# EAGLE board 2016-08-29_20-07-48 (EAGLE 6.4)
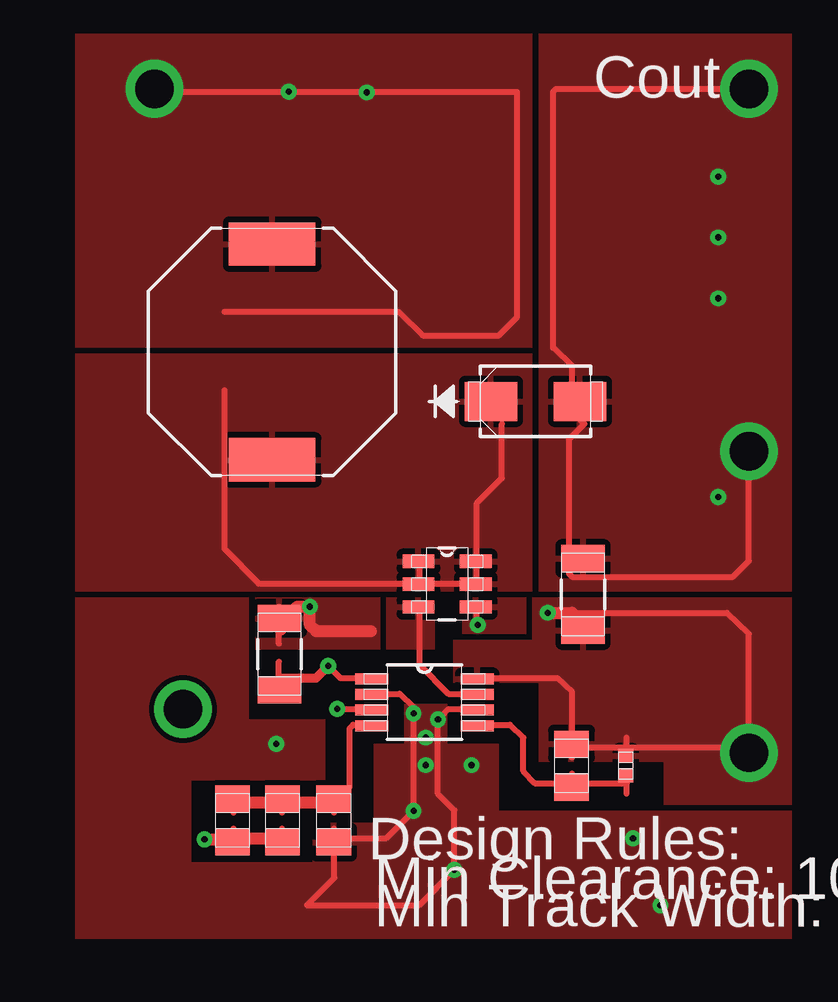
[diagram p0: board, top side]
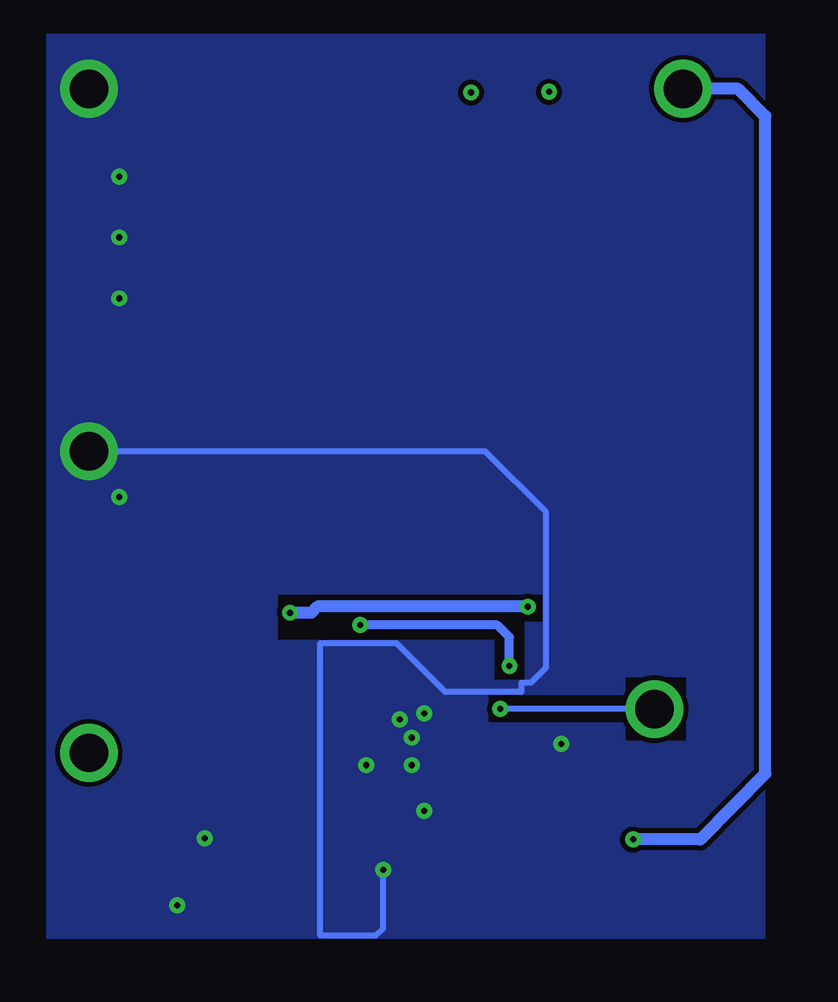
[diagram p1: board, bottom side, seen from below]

No outline drawn. Coordinates in mm, seen from the top.
Copper layers ((1*2)+(15*16)): TOP / INTERNAL1 / layer 15 / BOTTOM

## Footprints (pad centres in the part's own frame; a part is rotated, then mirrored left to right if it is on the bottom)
0805 = smd 1.118 x 1.448: 1 -0.902,0; 2 0.902,0
1206 = smd 1.118 x 1.803: 1 -1.499,0; 2 1.499,0
SMA = smd 2.184 x 1.626: 1 -1.854,0; 2 1.854,0
TP-1502 = drill 0.813 round: 1 0,0
SRU1038 = smd 1.803 x 3.607: 1 -4.496,0; 2 4.496,0
SOT-23-6 = smd 1.321 x 0.559: 1 -1.194,0.95; 2 -1.194,0; 3 -1.194,-0.95; 4 1.194,-0.95; 5 1.194,0; 6 1.194,0.95
0402 = smd 0.559 x 0.61: 1 -0.419,0; 2 0.419,0
MUA08A = smd 1.372 x 0.457: 1 -2.197,0.975; 2 -2.197,0.325; 3 -2.197,-0.325; 4 -2.197,-0.975; 5 2.197,-0.975; 6 2.197,-0.325; 7 2.197,0.325; 8 2.197,0.975

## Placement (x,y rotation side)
Cadj  [0805]  46.96,33.25 270 top
Cff  [0805]  32.84,30.96 90 top
Cin  [1206]  47.45,40.39 90 top
D1  [SMA]  45.47,48.44 0 top
GND  [TP-1502]  54.31,46.33 270 top
GND1  [TP-1502]  54.31,61.42 270 top
L1  [SRU1038]  34.49,50.5 90 top
M1  [SOT-23-6]  41.78,40.82 0 top
NC1  [TP-1502]  30.73,35.56 270 top
Radj  [0402]  49.23,33.25 270 top
Rfbb  [0805]  37.06,30.96 270 top
Rfbt  [0805]  34.92,30.96 90 top
Rsns  [1206]  34.8,37.9 90 top
U1  [MUA08A]  40.84,35.89 0 top
VIN  [TP-1502]  54.31,33.73 270 top
VOUT  [TP-1502]  29.54,61.42 270 top

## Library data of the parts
Cadj = ultra-librarian; RefDes: Cadj; Type: CL21C102JBCNFNC
Cff = ultra-librarian; RefDes: Cff; Type: CL21C331JBANFNC
Cin = ultra-librarian; RefDes: Cin; Type: GRM31CR71H475KA12L
D1 = ultra-librarian; RefDes: D1; Type: B340A-13-F
GND = ultra-librarian; RefDes: GND; Type: TP-1502
GND1 = ultra-librarian; RefDes: GND1; Type: TP-1502
L1 = ultra-librarian; RefDes: L1; Type: SRU1038-100Y
M1 = ultra-librarian; RefDes: M1; Type: FDC5614P
NC1 = ultra-librarian; RefDes: NC1; Type: TP-1502
Radj = ultra-librarian; RefDes: Radj; Type: CRCW040266K5FKED
Rfbb = ultra-librarian; RefDes: Rfbb; Type: ERJ-6ENF4322V
Rfbt = ultra-librarian; RefDes: Rfbt; Type: ERJ-6ENF4322V
Rsns = ultra-librarian; RefDes: Rsns; Type: CSR1206FK20L0
U1 = ultra-librarian; RefDes: U1; Type: LM3485MM/NOPB
VIN = ultra-librarian; RefDes: VIN; Type: TP-1502
VOUT = ultra-librarian; RefDes: VOUT; Type: TP-1502

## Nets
0: Cin.2 D1.2 GND1.1 GND.1 Rfbb.2 U1.2 U1.6
1: Cff.2 Rfbb.1 Rfbt.2 U1.4
2: Cadj.1 Cin.1 Radj.1 Rsns.2 U1.8 VIN.1
3: Cadj.2 Radj.2 U1.5
4: D1.1 L1.1 M1.1 M1.2 M1.5 M1.6
5: M1.4 Rsns.1 U1.1
6: Cff.1 L1.2 Rfbt.1 VOUT.1
7: M1.3 U1.7
8: NC1.1 U1.3

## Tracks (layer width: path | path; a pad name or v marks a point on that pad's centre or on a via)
0  (via drill 0.25 pad 0.56, 1.6 pad 2.21)
  TOP 0.254: v54.36,61.47 46.33,61.47 46.2,61.34 46.2,50.67 46.99,49.91 46.99,48.01 47.5,47.5 46.86,46.86 46.86,41.25 46.99,41.12 53.7,41.12 54.36,41.78 v54.36,46.35 | 38.73,36.25 39.8,36.25 40.39,35.69 v40.39,35.43 v40.39,31.37 39.24,30.23 37.08,30.23 37.08,28.57 35.94,27.43 40.62,27.43 v42.09,28.91 42.09,31.39 41.4,32.08 v41.4,35.18 | 43.03,35.61 41.83,35.61 41.53,35.31 41.53,35.18 | 37.07,29.79 37.07,30.63
  BOTTOM 0.254: v42.09,28.91 42.09,26.47 42.42,26.16 44.7,26.16 44.7,38.35 41.53,38.35 39.5,36.32 36.32,36.32 36.32,36.7 35.94,36.7 35.31,37.34 35.31,43.81 37.85,46.35 v54.36,46.35
  other vias: 53.09,57.81 53.09,55.27 53.09,52.73 53.09,44.45 50.67,27.43 34.67,34.16 40.89,33.27 49.53,30.23 42.8,33.27 40.89,34.42
  pour BOTTOM: 26.16,63.75 56.13,63.75 56.13,26.04 44.7,26.04 44.7,38.48 46.48,38.48 46.48,40.39 35.43,40.39 35.43,39.24 36.2,39.24 36.2,36.2 35.43,36.2 32,36.2 32,36.96 29.46,36.96 29.46,34.29 32,34.29 32,35.05 37.72,35.05 37.72,36.2 36.32,36.2 36.32,36.83 37.47,36.83 37.47,38.48 44.58,38.48 44.58,26.04 26.16,26.04
  pour TOP: 33.53,40.26 26.29,40.26 26.29,26.04 56.13,26.04 56.13,31.37 43.94,31.37 43.94,34.16 41.78,34.16 41.78,35.81 40.01,35.81 40.01,34.16 38.73,34.16 38.73,30.86 36.2,30.86 36.2,29.21 31.11,29.21 31.11,32.64 36.7,32.64 36.7,35.18 33.53,35.18
  pour TOP: 45.59,63.75 45.59,40.51 56.13,40.51 56.13,63.75
1
  TOP 0.254: 38.73,34.95 37.87,34.95 37.72,34.8 37.72,32.36 37.08,31.73 | 32.88,31.29 32.88,32.13 | 34.91,31.29 34.91,32.13 | 37.07,31.29 37.07,32.13
  TOP 0.508: 37.08,31.73 34.92,31.73 32.89,31.73
2  (via drill 0.25 pad 0.56, 1.6 pad 2.21)
  TOP 0.254: 46.99,39.62 53.44,39.62 54.36,38.73 v54.36,33.78 54.1,34.01 49.28,34.01 46.99,34.01 46.99,36.32 46.38,36.91 43.03,36.91 43.05,36.91 | 34.77,38.33 34.77,39.88 | 49.26,33.58 49.26,34.42 | 46.98,33.58 46.98,34.42 | v45.97,39.62
  TOP 0.508: 38.61,38.86 36.32,38.86 36.07,39.12 v36.07,39.88 35.56,39.88 34.85,39.17 34.85,38.91 | v45.97,39.62 46.99,39.62
  BOTTOM 0.508: v36.07,39.88 44.83,39.88 45.09,39.62 v45.97,39.62
  pour TOP (rank 3): 45.59,33.4 45.59,36.7 42.04,36.7 42.04,38.48 45.34,38.48 45.34,40.26 56.13,40.26 56.13,31.62 50.8,31.62 50.8,33.4
  pour TOP (rank 5): 33.78,40.26 38.99,40.26 38.99,38.1 33.78,38.1
3
  TOP 0.254: 49.28,32.51 46.99,32.51 45.44,32.51 44.96,33.02 44.96,34.42 44.4,34.95 43.03,34.95 | 49.26,32.08 49.26,32.92 | 46.98,32.08 46.98,32.92
4
  TOP 0.254: 32.51,48.9 32.51,42.29 33.93,40.84 40.64,40.84 | 40.64,40.84 40.64,41.78 | 40.64,40.84 43.03,40.84 | 44.07,47.5 44.07,45.24 43.03,44.2 43.03,40.89 | 42.65,41.77 43.38,41.77 | 42.65,40.83 43.38,40.83 | 40.26,40.83 41,40.83 | 40.26,41.77 41,41.77
  pour TOP (rank 4): 26.29,40.51 45.34,40.51 45.34,50.42 26.29,50.42
5  (via drill 0.25 pad 0.56)
  TOP 0.254: 34.8,36.96 34.82,36.91 | 37.34,36.91 | v36.83,37.41 37.34,36.91 | 37.34,36.91 38.73,36.91 | 43.03,39.9 43.03,39.12 v43.05,39.12 | 34.77,36.04 34.77,37.59 | 42.65,39.89 43.38,39.89
  TOP 0.381: 34.82,36.91 36.32,36.91 v36.83,37.41
  BOTTOM 0.381: v43.05,39.12 37.34,39.12 36.83,38.61 v36.83,37.41
  pour TOP: 42.42,40.26 42.42,38.73 45.09,38.73 45.09,40.26
6  (via drill 0.25 pad 0.56, 1.6 pad 2.21)
  TOP 0.254: v29.59,61.47 29.72,61.34 v35.18,61.34 44.7,61.34 44.7,61.32 44.7,51.94 43.94,51.18 40.77,51.18 39.75,52.17 32.51,52.17 | 32.84,30.18 32.89,30.23 | 32.88,29.79 32.88,30.63 | 34.91,29.79 34.91,30.63
  TOP 0.508: 32.89,30.23 34.92,30.23 | v31.67,30.18 32.84,30.18
  BOTTOM 0.254: v31.67,30.18 31.8,30.18
  BOTTOM 0.508: v29.59,61.47 27.3,61.47 26.16,60.33 26.16,32.92 28.88,30.18 v31.67,30.18
  other vias: 38.43,61.32
  pour TOP (rank 2): 26.29,50.67 45.34,50.67 45.34,63.75 26.29,63.75
7
  TOP 0.254: 43.03,36.25 41.83,36.25 40.64,37.44 40.64,39.9 | 40.26,39.89 41,39.89
  pour TOP (rank 6): 39.24,40.26 39.24,38.1 41.27,38.1 41.27,40.26
8  (via drill 0.25 pad 0.56, 1.6 pad 2.21)
  TOP 0.254: v37.21,35.61 38.73,35.61
  BOTTOM 0.254: v30.79,35.61 v37.21,35.61

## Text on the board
ASSYNOTES: Cout | Design Rules: | Min Clearance: 10mil | Min Track Width: 10mil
